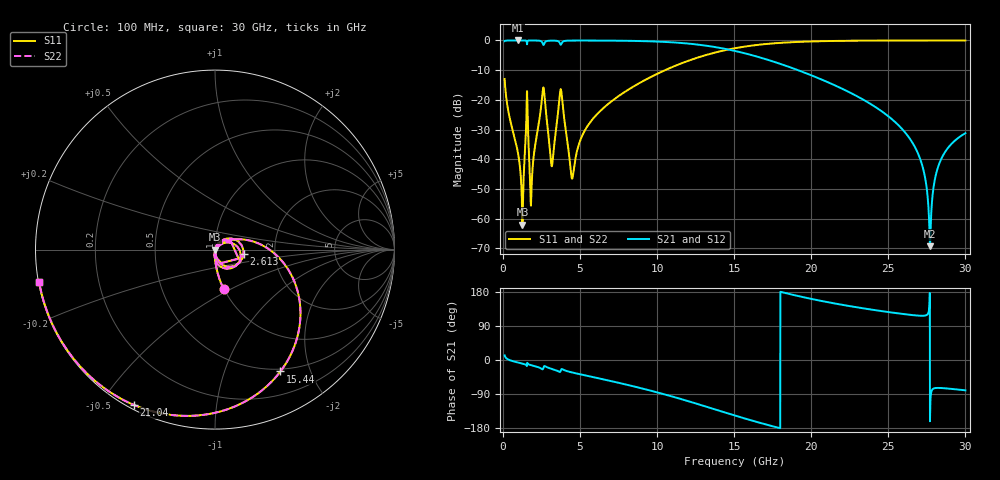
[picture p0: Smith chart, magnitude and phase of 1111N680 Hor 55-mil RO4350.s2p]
# GHz S MA R 50
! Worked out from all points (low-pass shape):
!   3201 points, 100 MHz to 30 GHz, reference 50 ohm
!   highest |S21| = -0.01 dB at 969 MHz (marker M1); lowest = -69.2 dB at 27.7 GHz (marker M2)
!   |S21| within 3 dB of the highest: start of sweep to 14.57 GHz
!   lowest |S11| = -61.9 dB at 1.259 GHz (marker M3), VSWR 1.00, Z = 50.1 - j0.00426 ohm
!   |S11| at or under -10 dB: start of sweep to 10.51 GHz
!   |S22| runs from -61.9 to 0.0 dB; largest |S21 - S12| = 0
!   S11 on the Smith chart (normalised r, x): 100 MHz: 0.99, -0.46; 2.613 GHz: 1.38, -0.07; 15.44 GHz: 0.47, -1.57; 21.04 GHz: 0.02, -0.61; 30 GHz: 0.00, -0.09
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0.1  0.2247 -77.7  0.9742 12.2  0.9742 12.2  0.2247 -77.7
0.9689688  0.01273 -94.2  0.9993 -6.5  0.9993 -6.5  0.01273 -94.2
1.258625  0.0008006 -3.0  0.9991 -9.4  0.9991 -9.4  0.0008006 -3.0
1.510906  0.0479 59.1  0.9848 -13.9  0.9848 -13.9  0.0479 59.1
1.865969  0.004242 53.9  0.9982 -14.1  0.9982 -14.1  0.004242 53.9
2.613469  0.1618 -9.3  0.8409 -21.4  0.8409 -21.4  0.1618 -9.3
3.146063  0.00774 -28.6  0.9919 -23.3  0.9919 -23.3  0.00774 -28.6
3.734719  0.1509 -20.1  0.8502 -28.9  0.8502 -28.9  0.1509 -20.1
4.454187  0.004873 -39.7  0.9947 -32.7  0.9947 -32.7  0.004873 -39.7
5.089563  0.02352 44.1  0.9961 -38.5  0.9961 -38.5  0.02352 44.1
6.75275  0.0825 35.0  0.9933 -53.3  0.9933 -53.3  0.0825 35.0
10.06978  0.2798 3.2  0.9558 -86.2  0.9558 -86.2  0.2798 3.2
15.05  0.74 -57.0  0.6654 -146.6  0.6654 -146.6  0.74 -57.0
15.44244  0.7706 -61.8  0.6299 -151.4  0.6299 -151.4  0.7706 -61.8
20.03956  0.9628 -109.4  0.2568 160.9  0.2568 160.9  0.9628 -109.4
21.03934  0.9763 -117.6  0.2001 152.8  0.2001 152.8  0.9763 -117.6
25.01978  0.9956 -144.3  0.05251 126.4  0.05251 126.4  0.9956 -144.3
26.95394  0.997 -154.9  0.01204 117.1  0.01204 117.1  0.997 -154.9
27.36506  0.997 -157.0  0.005221 117.1  0.005221 117.1  0.997 -157.0
27.70144  0.997 -158.7  0.0003458 -161.6  0.0003458 -161.6  0.997 -158.7
28.37419  0.997 -162.0  0.009389 -73.8  0.009389 -73.8  0.997 -162.0
30  0.9966 -169.6  0.02749 -80.0  0.02749 -80.0  0.9966 -169.6
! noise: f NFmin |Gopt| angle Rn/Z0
0.1  0.0006435  0.7268  1.429  0.0004683
3.417  0.02508  0.7596  25.21  0.02015
6.743  0.01809  0.471  47.08  0.004988
10.06  0.02508  0.4636  64.59  0.005933
13.39  0.03678  0.532  80.26  0.008642
16.7  0.05844  0.6523  97.15  0.01479
20.03  0.1072  0.7909  116.2  0.03054
23.35  0.2539  0.9062  135.6  0.08613
26.67  1.489  0.983  153.6  1.07
30  0.9465  0.9727  169.5  0.0676
